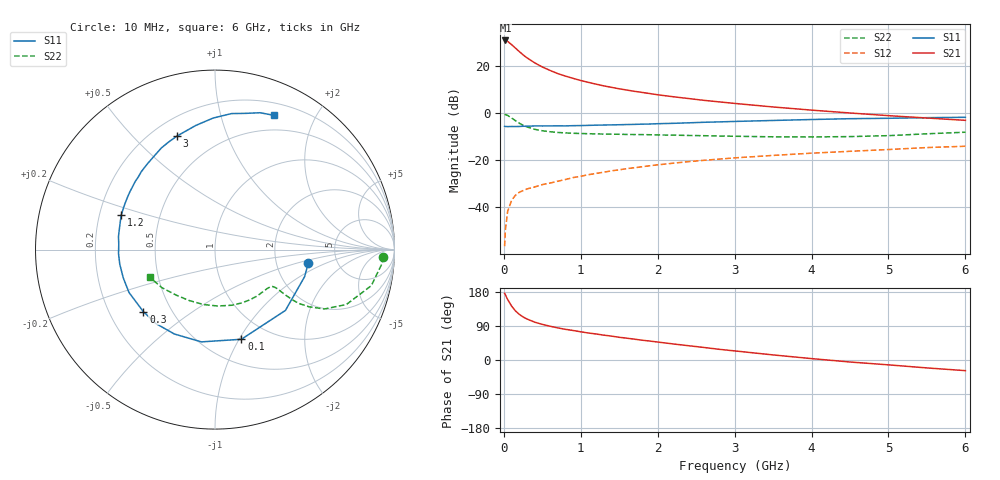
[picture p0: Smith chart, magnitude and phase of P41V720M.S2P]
! SIEMENS Small Signal Semiconductors
! BFP182
! Si NPN RF Bipolar Junction Transistor in SOT143
! VCE = 1.75 V  IC = 20 mA
! Common Emitter S-Parameters:  March  1996
# GHz  S  MA  R  50
!  f  S11  S21  S12  S22
! GHz  MAG  ANG  MAG  ANG  MAG  ANG  MAG  ANG
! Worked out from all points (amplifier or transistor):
!   36 points, 10 MHz to 6 GHz, reference 50 ohm
!   highest |S21| = 30.9 dB at 20 MHz (marker M1)
!   |S21| within 3 dB of that: start of sweep to 142.3 MHz
!   unconditionally stable (mu >= 1): 553.5 MHz to end of sweep
!   at 250 MHz: K = 0.60, MSG = 28.8 dB, |S12| = -32.9 dB
!   at 1.4 GHz: K = 1.31, MAG = 14.4 dB, |S12| = -24.5 dB
!   at 6 GHz: K = 1.02, MAG = 4.7 dB, |S12| = -14.1 dB
!   S11 on the Smith chart (normalised r, x): 10 MHz: 3.06, -0.65; 100 MHz: 0.75, -1.02; 300 MHz: 0.35, -0.33; 1.2 GHz: 0.29, +0.16; 3 GHz: 0.30, +0.68; 6 GHz: 0.33, +1.48
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0.01  0.5252 -8.4  34.83 175.8  0.0015 81.8  0.9364 -2.4
0.02  0.5215 -16.8  34.98 171.9  0.0033 80.5  0.9311 -5.2
0.05  0.5185 -40.8  33.34 159.4  0.0083 76.1  0.8938 -13.0
0.1  0.5208 -73.6  28.62 142.6  0.014 61.7  0.7931 -22.7
0.15  0.5197 -98.4  24.12 129.8  0.018 54.8  0.6934 -28.5
0.2  0.5219 -115.7  20.39 120.6  0.0209 50.7  0.6136 -31.3
0.25  0.5274 -128.6  17.32 113.6  0.0227 48.7  0.5554 -32.7
0.3  0.5281 -139.1  15 108.3  0.0246 47.2  0.5111 -33.0
0.4  0.5354 -153.5  11.75 99.9  0.0271 47.8  0.4544 -32.7
0.5  0.5348 -162.9  9.558 94.0  0.0304 48.3  0.4232 -32.3
0.6  0.5367 -171.2  8.098 89.1  0.0328 49.6  0.4034 -32.1
0.7  0.538 -177.6  6.927 84.8  0.0359 51.4  0.3898 -32.3
0.8  0.537 176.8  6.13 81.0  0.039 51.9  0.3809 -32.7
1.1  0.5508 163.2  4.506 71.2  0.0494 53.6  0.3663 -35.5
1.2  0.5567 159.6  4.126 68.6  0.0526 53.8  0.3626 -36.8
1.6  0.5735 145.7  3.095 57.5  0.0664 53.2  0.3533 -42.9
2.2  0.6083 128.3  2.233 42.4  0.0866 49.9  0.3419 -54.4
3  0.667 108.6  1.611 24.0  0.1123 43.4  0.3234 -73.5
3.5  0.6999 98.8  1.354 13.4  0.1268 39.0  0.3146 -87.3
4.5  0.7633 83.1  1.009 -5.3  0.155 30.4  0.318 -116.8
5.5  0.8027 71.8  0.789 -20.9  0.1862 21.8  0.3648 -144.6
6  0.8168 66.4  0.704 -28.1  0.1983 16.6  0.3943 -157.1
